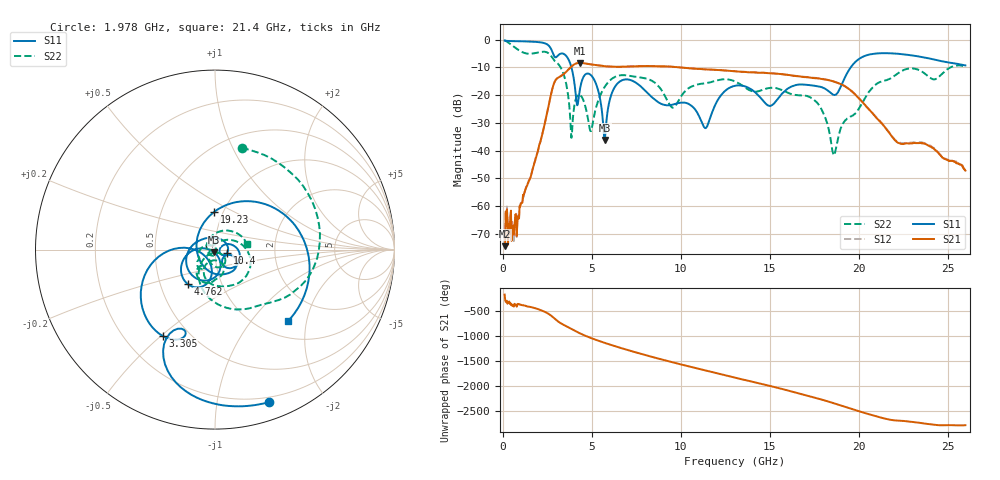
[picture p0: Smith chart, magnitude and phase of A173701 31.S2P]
!  2-Port S-parameters saved by WinCal
! VAR MeasName=S-Parameters (CALIBRATED_DATA) read from VNA (N5245A)
! VAR MeasDate=2017-6-7 10:30:25
! VAR NAME=A173701 31
! VAR FILENAME=A173701 31.S2P
! VAR DATE=2017-6-7 10:30:25
! VAR PHYS_PORTS=1,2
# Hz S DB R 50
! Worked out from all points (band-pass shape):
!   801 points, 100 MHz to 26 GHz, reference 50 ohm
!   highest |S21| = -8.39 dB at 4.341 GHz (marker M1); lowest = -74.4 dB at 100 MHz (marker M2)
!   |S21| within 3 dB of the highest: 3.595 GHz to 13 GHz (9.4 GHz wide, 113 % of centre)
!   lowest |S11| = -36.1 dB at 5.733 GHz (marker M3), VSWR 1.03, Z = 49.4 - j1.42 ohm
!   |S11| at or under -10 dB: 3.855 GHz to 19.56 GHz (15.7 GHz wide, 134 % of centre)
!   |S22| runs from -41.7 to -0.3 dB; largest |S21 - S12| = 0.0039
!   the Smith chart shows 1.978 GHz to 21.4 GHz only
!   S11 on the Smith chart (normalised r, x): 1.978 GHz: 0.15, -1.41; 3.305 GHz: 0.36, -0.51; 4.762 GHz: 0.69, -0.28; 10.4 GHz: 1.15, -0.04; 19.23 GHz: 0.91, +0.40; 21.4 GHz: 1.32, -1.56
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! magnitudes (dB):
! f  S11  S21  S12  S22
! 100 MHz  -0.3  -74.4  -72.5  -0.3
! 682.8 MHz  -0.6  -65.1  -65.2  -2.9
! 1.978 GHz  -0.9  -40.0  -40.0  -4.6
! 3.305 GHz  -5.0  -13.0  -13.0  -10.7
! 3.856 GHz  -10.0  -9.7  -9.7  -35.4
! 4.341 GHz  -17.6  -8.4  -8.4  -19.9
! 4.438 GHz  -15.0  -8.4  -8.4  -20.7
! 4.762 GHz  -12.2  -8.7  -8.7  -27.7
! 5.733 GHz  -36.1  -9.6  -9.6  -16.9
! 6.672 GHz  -14.7  -9.8  -9.8  -12.8
! 8.744 GHz  -22.6  -9.6  -9.6  -16.8
! 9.553 GHz  -23.4  -9.8  -9.8  -24.5
! 10.4 GHz  -23.0  -10.3  -10.3  -17.7
! 11.4 GHz  -31.9  -10.8  -10.7  -15.7
! 13.05 GHz  -16.6  -11.4  -11.4  -15.1
! 15.02 GHz  -23.9  -12.1  -12.1  -17.4
! 17.39 GHz  -16.5  -13.8  -13.7  -21.2
! 18.62 GHz  -20.0  -15.1  -15.1  -41.7
! 19.23 GHz  -13.6  -16.8  -16.9  -29.2
! 21.4 GHz  -4.9  -31.0  -30.9  -14.9
! 21.69 GHz  -4.9  -33.4  -33.2  -14.3
! 26 GHz  -9.3  -47.2  -47.0  -9.9
